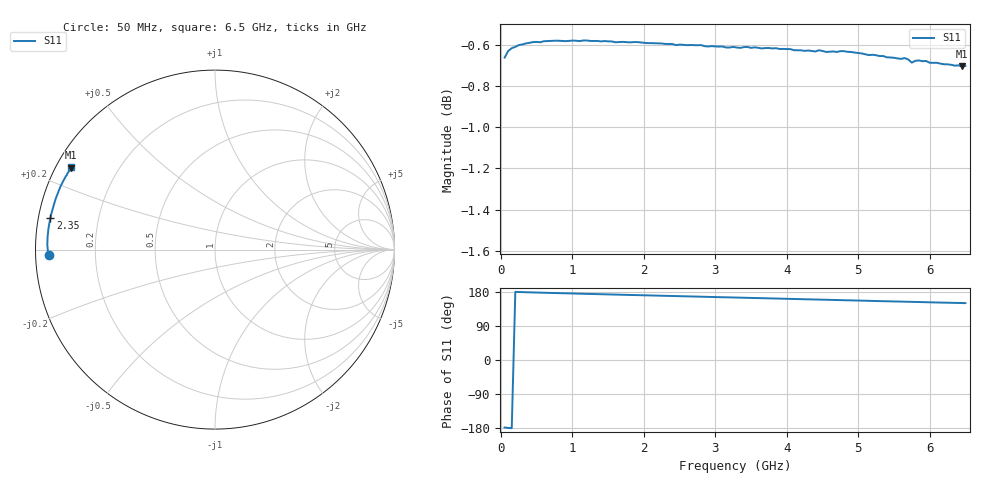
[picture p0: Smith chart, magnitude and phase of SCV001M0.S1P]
! Infineon Technologies  Discrete & RF Semiconductors
! BAR63-02L
! Si PIN Diode in TSLP-2
! IF = 1 mA
! S-Parameters:  March  2002
# GHz  S  MA  R  50
!  f  S11
! GHz  MAG  ANG
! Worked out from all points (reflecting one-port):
!   130 points, 50 MHz to 6.5 GHz, reference 50 ohm
!   lowest |S11| = -0.7 dB at 6.45 GHz (marker M1), VSWR 24.70, Z = 2.17 + j13.2 ohm
!   phase of S11 starts at -178 deg and turns -32 deg over the sweep
!   S11 on the Smith chart (normalised r, x): 50 MHz: 0.04, -0.02; 2.35 GHz: 0.03, +0.10; 6.5 GHz: 0.04, +0.27
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0.05  0.9267 -178.1
0.1  0.9301 -179.3
0.15  0.9316 -179.8
0.25  0.9332 179.4
0.4  0.9344 178.5
0.9  0.9353 176.0
1.2  0.9356 174.5
1.7  0.9349 172.2
2.35  0.9338 169.1
2.45  0.9332 168.7
2.5  0.9335 168.4
2.9  0.9325 166.6
2.95  0.9327 166.3
3.1  0.9325 165.7
3.3  0.9319 164.7
3.75  0.9317 162.7
4.1  0.9305 161.0
4.25  0.9302 160.4
4.3  0.9304 160.1
4.4  0.9299 159.7
4.45  0.9305 159.4
4.55  0.9296 159.0
4.9  0.9296 157.3
5.3  0.9275 155.4
5.65  0.9264 153.9
5.7  0.9257 153.6
6.45  0.9222 150.3
6.5  0.9223 150.1
